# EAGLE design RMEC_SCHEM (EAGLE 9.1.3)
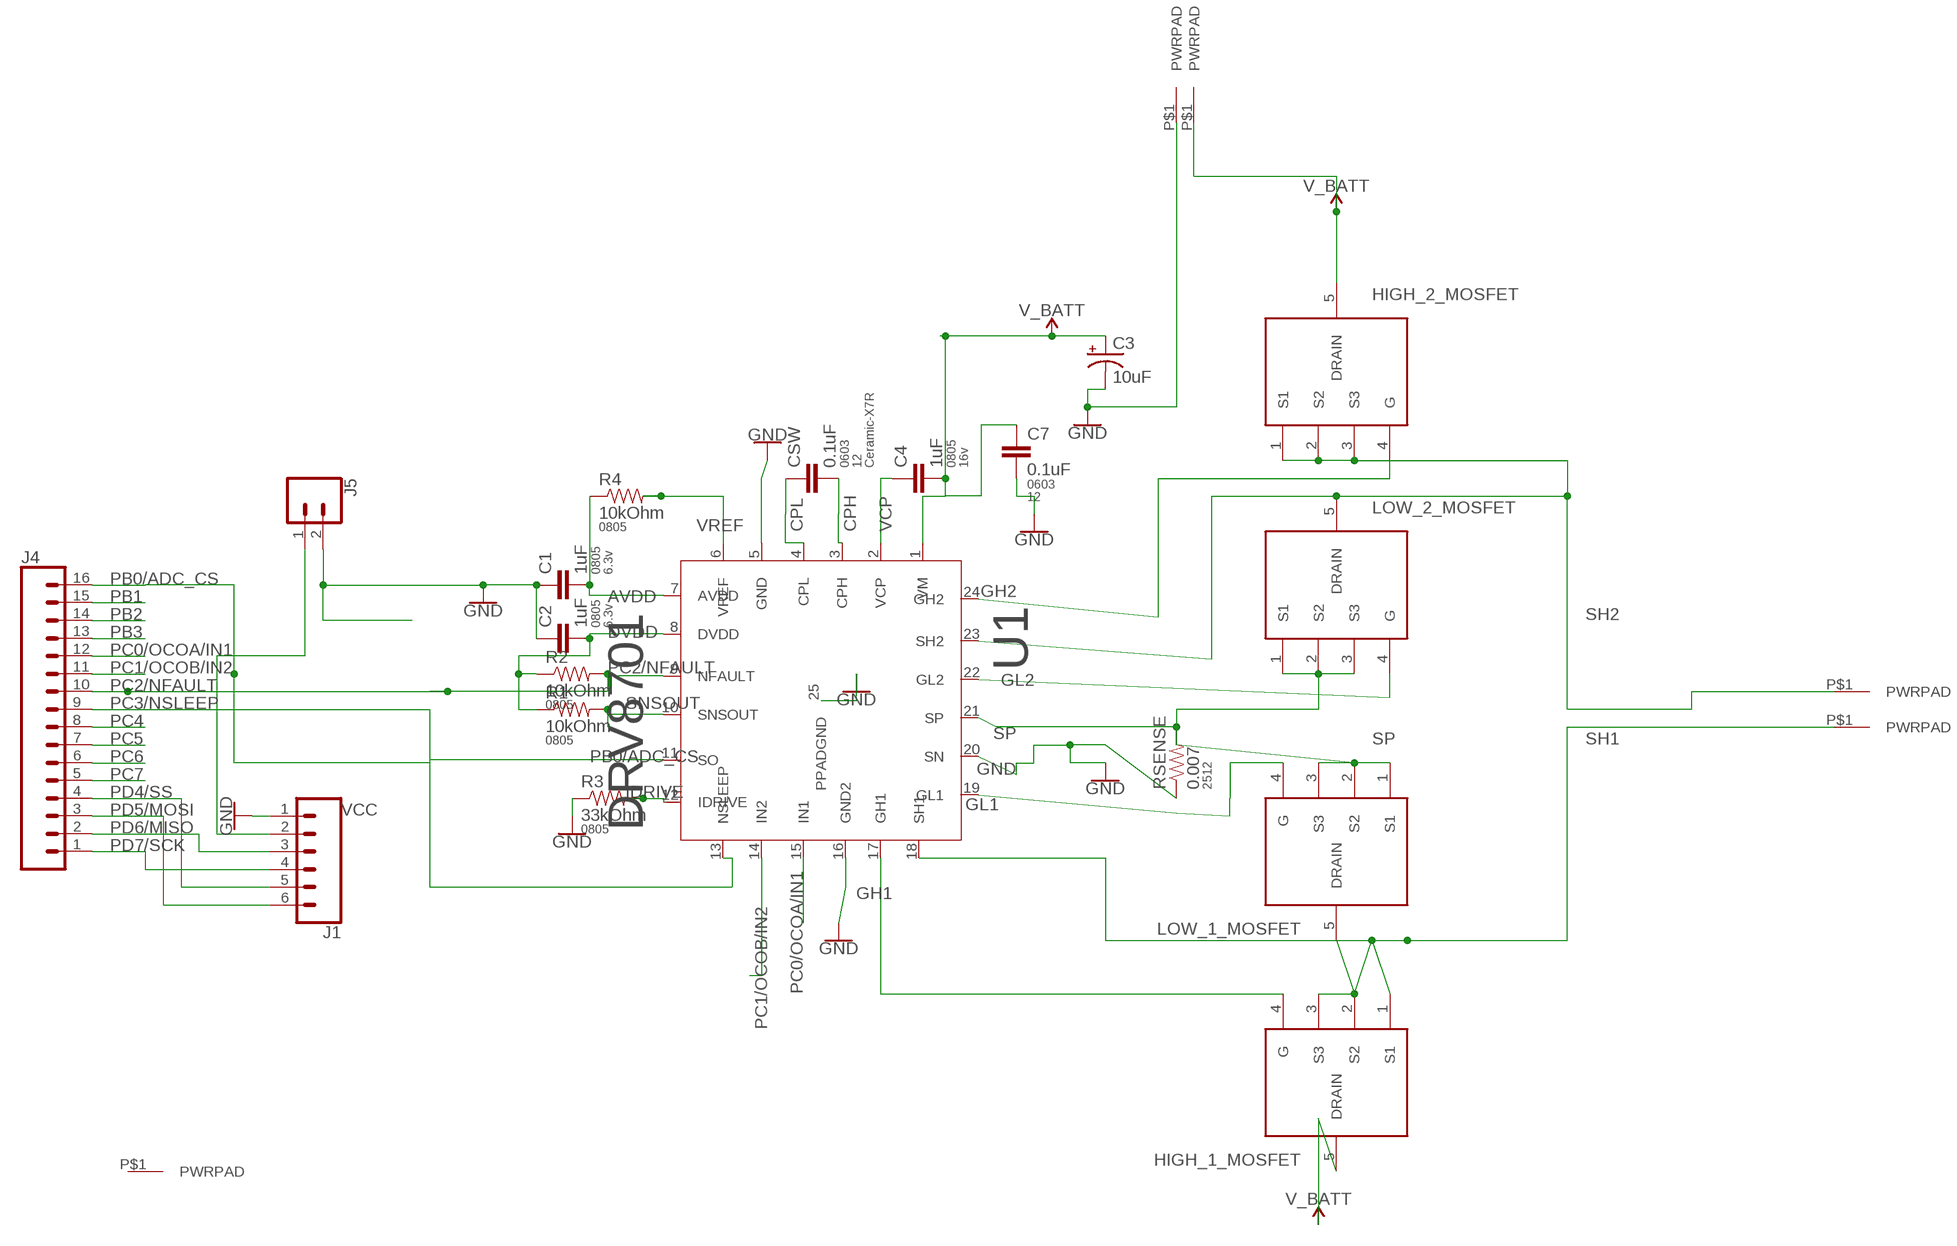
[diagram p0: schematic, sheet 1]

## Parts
C1  1uF  CAP0805  [0805]
C2  1uF  CAP0805  [0805]
C3  10uF  10UF-POLAR-RADIAL-2.5MM-25V-20%  [CPOL-RADIAL-2.5MM-5MM]
C4  1uF  CAP0805  [0805]
C7  0.1uF  CAP0603-CAP  [0603-CAP]
CSW  0.1uF  CAP0603-CAP  [0603-CAP]
GND  PWRPADM3-STANDOFF  [PWRPAD_M3_STANDOFF]
HIGH_1_MOSFET  AON7410  [AON7410]
HIGH_2_MOSFET  AON7410  [AON7410]
J1  CONN_06NO_SILK_FEMALE_PTH  [1X06_NO_SILK]
J3  PWRPADM3  [PWRPAD_3-25MM]
J4  CONN_16  [1X16]
J5  CONN_02  [1X02]
J6  PWRPADM3-STANDOFF  [PWRPAD_M3_STANDOFF]
J7  PWRPADM3-STANDOFF  [PWRPAD_M3_STANDOFF]
LOW_1_MOSFET  AON7410  [AON7410]
LOW_2_MOSFET  AON7410  [AON7410]
R1  10kOhm  RESISTOR0805-RES  [0805]
R2  10kOhm  RESISTOR0805-RES  [0805]
R3  33kOhm  RESISTOR0805-RES  [0805]
R4  10kOhm  RESISTOR0805-RES  [0805]
RSENSE  0.007  RESISTOR2512  [R2512]
U1  DRV8701  [DRV8701]
VM  PWRPADM3-STANDOFF  [PWRPAD_M3_STANDOFF]

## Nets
AVDD: C1.2 R4.1 U1.7(AVDD)
CPH: CSW.2 U1.3(CPH)
CPL: CSW.1 U1.4(CPL)
DVDD: C2.2 R1.1 R2.1 U1.8(DVDD)
GH1: HIGH_1_MOSFET.4(G) U1.17(GH1)
GH2: HIGH_2_MOSFET.4(G) U1.24(GH2)
GL1: LOW_1_MOSFET.4(G) U1.19(GL1)
GL2: LOW_2_MOSFET.4(G) U1.22(GL2)
GND: C1.1 C2.1 C3.2(-) C7.2 GND.P$1(PWRPAD) J1.1 J5.2 R3.1 RSENSE.1 U1.5(GND) U1.16(GND2) U1.20(SN) U1.25(PPADGND)
IDRIVE: R3.2 U1.12(IDRIVE)
PB0/ADC_CS: J4.16 U1.11(SO)
PB1: J4.15
PB2: J4.14
PB3: J4.13
PC0/OCOA/IN1: J4.12 U1.15(IN1)
PC1/OCOB/IN2: J4.11 U1.14(IN2)
PC2/NFAULT: J4.10 R2.2 U1.9(NFAULT)
PC3/NSLEEP: J4.9 U1.13(NSLEEP)
PC4: J4.8
PC5: J4.7
PC6: J4.6
PC7: J4.5
PD4/SS: J1.5 J4.4
PD5/MOSI: J1.6 J4.3
PD6/MISO: J1.3 J4.2
PD7/SCK: J1.4 J4.1
SH1: HIGH_1_MOSFET.1(S1) HIGH_1_MOSFET.2(S2) HIGH_1_MOSFET.3(S3) J7.P$1(PWRPAD) LOW_1_MOSFET.5(DRAIN) U1.18(SH1)
SH2: HIGH_2_MOSFET.1(S1) HIGH_2_MOSFET.2(S2) HIGH_2_MOSFET.3(S3) J6.P$1(PWRPAD) LOW_2_MOSFET.5(DRAIN) U1.23(SH2)
SNSOUT: R1.2 U1.10(SNSOUT)
SP: LOW_1_MOSFET.1(S1) LOW_1_MOSFET.2(S2) LOW_1_MOSFET.3(S3) LOW_2_MOSFET.1(S1) LOW_2_MOSFET.2(S2) LOW_2_MOSFET.3(S3) RSENSE.2 U1.21(SP)
V_BATT: C3.1(+) C4.2 C7.1 HIGH_1_MOSFET.5(DRAIN) HIGH_2_MOSFET.5(DRAIN) U1.1(VM) VM.P$1(PWRPAD)
VCC: J1.2 J5.1
VCP: C4.1 U1.2(VCP)
VREF: R4.2 U1.6(VREF)
Unconnected: J3.P$1(PWRPAD)

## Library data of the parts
C1 C2 = passives:CAP: Capacitor; PACKAGE: 0805; VOLTAGE: 6.3v
C3 = SparkFun-Capacitors:10UF-POLAR: 10.0µF polarized capacitors; PROD_ID: CAP-08440
C4 = passives:CAP: Capacitor; PACKAGE: 0805; VOLTAGE: 16v
C7 = passives:CAP: Capacitor; PACKAGE: 0603; VOLTAGE: 12
CSW = passives:CAP: Capacitor; PACKAGE: 0603; TYPE: Ceramic-X7R; VOLTAGE: 12
GND J3 J6 J7 VM = power:PWRPAD
HIGH_1_MOSFET HIGH_2_MOSFET LOW_1_MOSFET LOW_2_MOSFET = RCustom:AON7410
J1 = SparkFun-Connectors:CONN_06: Multi connection point. Often used as Generic Header-pin footprint for 0.1 inch spaced/style header connections On any of the 0.1 inch spaced packages, you can populate with these: Break Away Headers - Straight (PRT-00116) Break Away Male Headers - Right Angle (PRT-00553) Female Headers (PRT-00115)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; PROD_ID: CONN-08437
J4 = SparkFun-Connectors:CONN_16: Multi connection point. Often used as Generic Header-pin footprint for 0.1 inch spaced/style header connections On any of the 0.1 inch spaced packages, you can populate with these: Break Away Headers - Straight (PRT-00116) Break Away Male Headers - Right Angle (PRT-00553) Female Headers (PRT-00115)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
J5 = SparkFun-Connectors:CONN_02: Multi connection point. Often used as Generic Header-pin footprint for 0.1 inch spaced/style header connections
R1-R4 = passives:RESISTOR: Resistor; PACKAGE: 0805
RSENSE = passives:RESISTOR: Resistor; PACKAGE: 2512
U1 = RCustom:DRV8701: This is the DRV8701, one of TI's gate drivers to make a full bridge for motor control. Includes current sense logic inside with an external sense resistor.

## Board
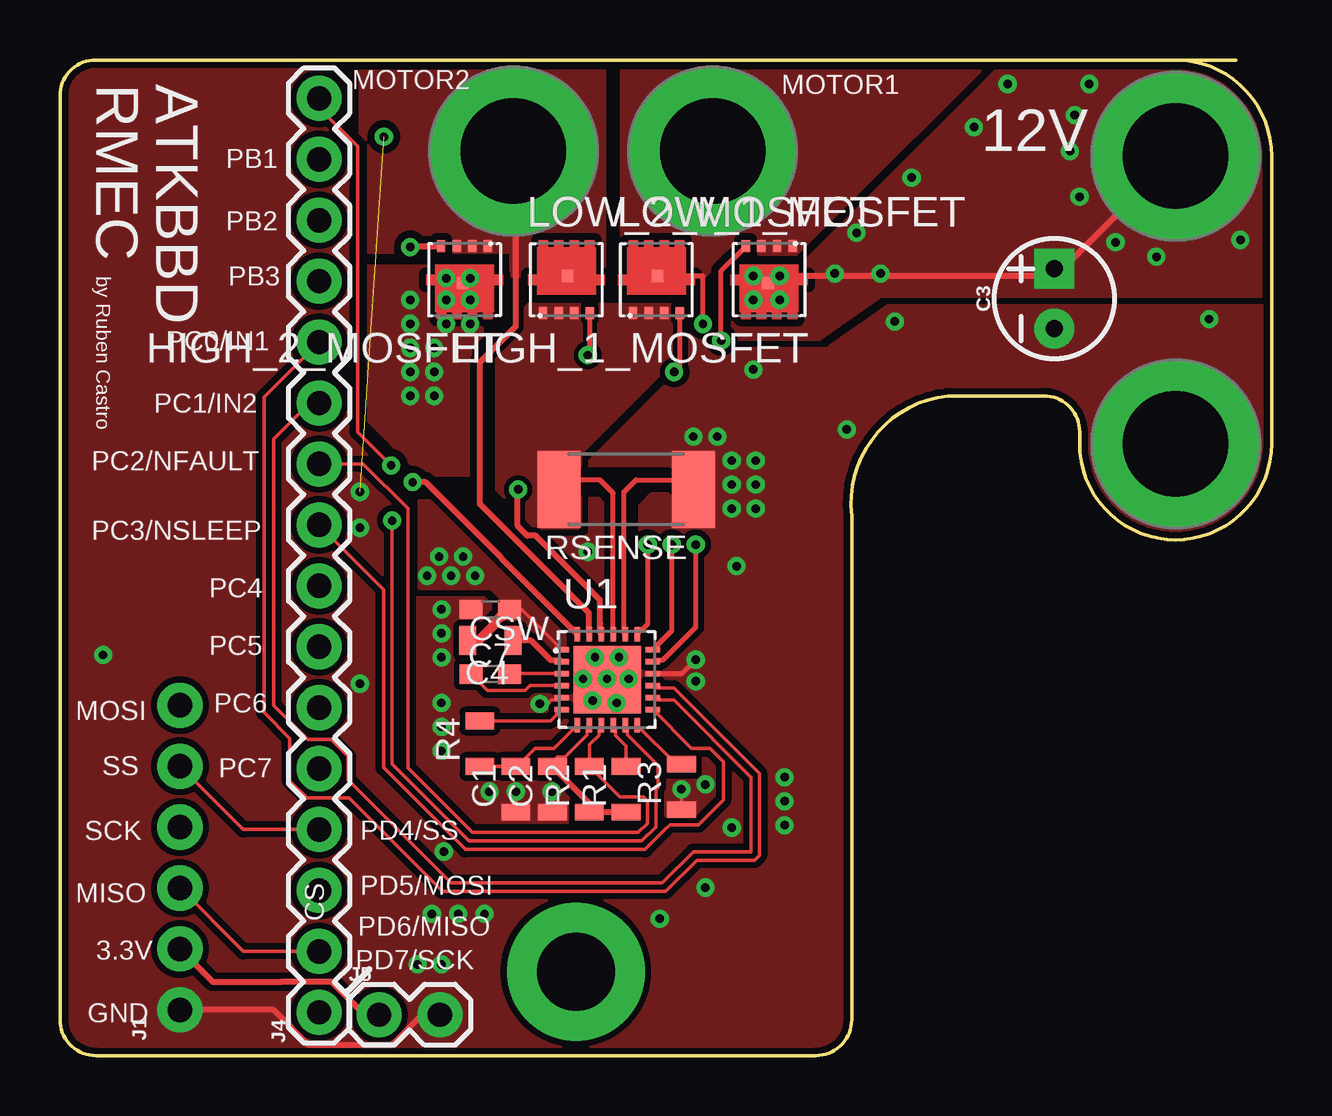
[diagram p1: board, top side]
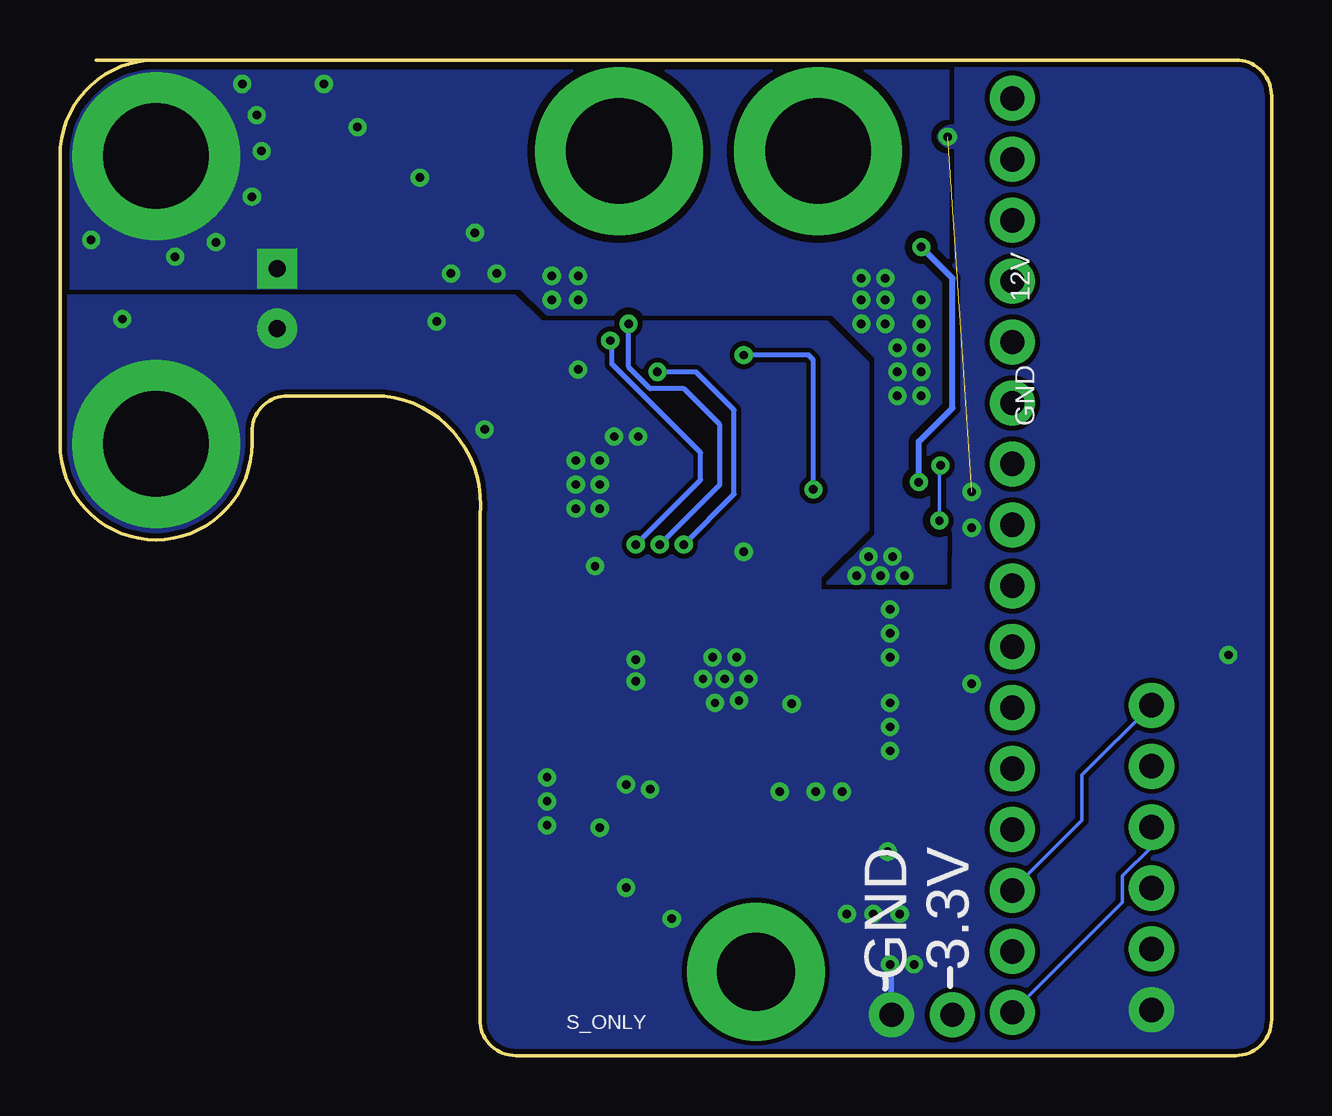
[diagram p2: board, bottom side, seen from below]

Size 50.5 x 41.5 mm. Coordinates in mm from the lower left corner, seen from the top.
Outline: 46.5,41.5 arc-90 50.5,37.5 50.5,25.5 arc-90 46.5,21.5 arc-90 42.5,25.5 42.5,26 arc90 41,27.5 37,27.5 arc90 33,22.5 33,1.5 arc-90 31.5,0 1.5,0 arc-90 0,1.5 0,40 arc-90 1.5,41.5 49,41.5
Copper layers (1*16): Top 0.035mm / dielectric 1.5mm / Bottom 0.035mm
Design rules "default *": minimum track width 6mil, minimum drill 0.35mm, track to track 8mil, track to pad 8mil, pad to pad 8mil, via to via 8mil, smd to smd 8mil, copper to edge 8mil, drill to drill 8mil, minimum pad ring 10mil, minimum via ring 8mil, stop-mask expansion 4mil, vias tented up to drill 25mil, thermal gap 10mil

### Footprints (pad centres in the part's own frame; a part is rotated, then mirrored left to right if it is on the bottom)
0805 = smd 0.7 x 1.2: 1 -0.95,0; 2 0.95,0
CPOL-RADIAL-2.5MM-5MM = drill 0.7 pad 1.651 square: 1 1.25,0 | drill 0.7 pad 1.651: 2 -1.25,0
0603-CAP = smd 0.96 x 0.8: 1 -0.8,0; 2 0.8,0
PWRPAD_M3_STANDOFF = drill 4.4 pad 7: P$1 0,0
AON7410 = smd 0.35 x 0.5: 1 -0.975,-1.4; 2 -0.325,-1.4; 3 0.325,-1.4; 4 0.975,-1.4 | smd 0.5 x 0.5: 5 0.05,0.15
1X06_NO_SILK = drill 1.016 pad 1.88: 1 0,0; 2 2.54,0; 3 5.08,0; 4 7.62,0; 5 10.16,0; 6 12.7,0
PWRPAD_3-25MM = drill 3.25 pad 5.75: P$1 0,0
1X16 = drill 1.016 pad 1.88: 1 0,0; 2 2.54,0; 3 5.08,0; 4 7.62,0; 5 10.16,0; 6 12.7,0; 7 15.24,0; 8 17.78,0; 9 20.32,0; 10 22.86,0; 11 25.4,0; 12 27.94,0; 13 30.48,0; 14 33.02,0; 15 35.56,0; 16 38.1,0
1X02 = drill 1.016 pad 1.88: 1 0,0; 2 2.54,0
R2512 = smd 1.8 x 3.2: 1 -2.8,0; 2 2.8,0
DRV8701 = smd 0.6 x 0.24: 1 -1.9,1.25; 2 -1.9,0.75; 3 -1.9,0.25; 4 -1.9,-0.25; 5 -1.9,-0.75; 6 -1.9,-1.25; 13 1.9,-1.25; 14 1.9,-0.75; 15 1.9,-0.25; 16 1.9,0.25; 17 1.9,0.75; 18 1.9,1.25 | smd 0.24 x 0.6: 7 -1.25,-1.9; 8 -0.75,-1.9; 9 -0.25,-1.9; 10 0.25,-1.9; 11 0.75,-1.9; 12 1.25,-1.9; 19 1.25,1.9; 20 0.75,1.9; 21 0.25,1.9; 22 -0.25,1.9; 23 -0.75,1.9; 24 -1.25,1.9 | smd 2.8 x 2.8: 25 0,0

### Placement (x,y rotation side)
C1  19,11.1 90 top
C2  20.53,11.1 90 top
C3  41.45,31.55 90 top
C4  17.94,17.3 180 top
C7  17.94,18.6 180 top
CSW  17.94,15.9 0 top
GND  46.5,25.5 0 top
HIGH_1_MOSFET  29.56,32.34 180 top
HIGH_2_MOSFET  16.86,32.34 180 top
J1  5,1.9 90 top
J3  21.5,3.5 0 top
J4  10.8,1.8 90 top
J5  13.3,1.7 0 top
J6  18.9,37.7 0 top
J7  27.2,37.7 0 top
LOW_1_MOSFET  24.86,32.34 0 top
LOW_2_MOSFET  21.11,32.34 0 top
R1  23.6,11.1 90 top
R2  22.07,11.1 90 top
R3  25.9,11.2 90 top
R4  17.5,13 90 top
RSENSE  23.6,23.6 180 top
U1  22.81,15.67 0 top
VM  46.5,37.5 0 top

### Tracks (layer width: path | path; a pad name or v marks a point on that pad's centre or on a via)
AVDD
  Top 0.152: U1.7 20.59,12.8 19.8,12.8 19.05,12.05 C1.2 R4.1
CLEAR
  cutout Top (isolate 0.305, no thermals): 22.8,17.5 23.6,17.5 24,17.9 24,23 24.6,23.6 25.4,23.6 25.5,23.5 25.5,24.3 25.4,24.4 21.7,24.4 21.7,23.7 21.7,23.4 22.5,23.4 22.8,23.1
CPH
  Top 0.152: U1.3 18.76,15.92 CSW.2
CPL
  Top 0.152: U1.4 19.59,15.42 19.4,15.22 17.82,15.22 CSW.1
CUTOFFGND
  cutout Top (rank 3, no thermals): 23.8,17.3 23.3,17.3 23.3,17.1 23.8,17.1
DVDD
  Top 0.152: C2.2 20.53,12.24 20.73,12.44 21.05,12.44 21.96,13.35 21.96,13.67 U1.8
  Top 0.254: C2.2 22.07,10.52 R2.1 R1.1
GH1  (via drill 0.35)
  Top 0.203: U1.17 24.79,16.5 25.14,16.5 26.5,17.86 v26.5,21.3 | v27.56,29.8 27.56,32.72 HIGH_1_MOSFET.4
  Bottom 0.203: v27.56,29.8 27.5,29.8 27.5,28.82 23.8,25.12 23.8,24 v26.5,21.3
GH2  (via drill 0.35)
  Top 0.254: U1.24 15.23,23.9 v14.7,23.9 | v14.6,33.7 14.64,33.74 HIGH_2_MOSFET.4
  Bottom 0.254: v14.7,23.9 14.7,25.6 13.3,27 13.3,32.4 v14.6,33.7
GL1  (via drill 0.35)
  Top 0.203: U1.19 24.5,18.01 v24.5,21.3 | v25.6,28.5 25.84,28.73 LOW_1_MOSFET.4
  Bottom 0.203: v24.5,21.3 22.4,23.4 22.4,26.9 24,28.5 v25.6,28.5
GL2  (via drill 0.35)
  Top 0.203: v22,29.2 22.09,29.29 LOW_2_MOSFET.4
  Top 0.254: U1.22 22.52,17.61 22.52,18 22.5,18.02 22.5,19 19.83,21.67 19.48,21.67 19.07,22.07 19.07,23.57 v19.1,23.6
  Bottom 0.203: v19.1,23.6 19.1,29 19.3,29.2 v22,29.2
GND  (via drill 0.35)  (1 unrouted)
  Top 0.152: U1.20 23.5,17.63 | C1.1 v19,11 | C2.1 20.5,10.18 v20.5,11 | v25.9,11.1 R3.1 | U1.5 20.81,14.82 20.49,14.82 20.34,14.66 v20,14.66
  Top 0.2: 24,24 26,24 RSENSE.1
  Top 0.203: 23.5,17.63 23.5,23.5 24,24 | U1.16 25.92,15.92 v26.5,16.5
  Top 0.254: J5.2 15.64,1.9 15.3,1.9 13.83,0.43 10.37,0.43 8.9,1.9 J1.1
  Bottom 0.254: J5.2 15.84,3.74 v15.9,3.8
  other vias: 21.8,15.7 22.2,14.8 23.2,14.7 23.7,15.7 22.8,15.7 22.3,16.6 23.3,16.6 15.9,18.6 26.4,25.8 27.4,25.8 28,24.8 29,24.8 28,23.8 29,23.8 28,22.8 29,22.8 15.5,5.9 16.6,5.9 17.7,5.9 14.9,3.8 17.9,11 15.9,16.6 15.9,17.6 26.9,11.3 30.2,11.6 30.2,10.6 30.2,9.6 26.5,15.6 15.9,14.7 15.9,13.7 15.9,12.7 22,21 28,9.5 16,8.5 12.5,15.5 12.5,22 12.5,23.5 34.8,30.6 47.9,30.7 32.8,26.1 28.9,28.6 26.9,7 28.2,20.4 25,5.7 1.8,16.7 13.5,38.3
  pour Bottom (rank 3, no thermals): -1,54 -4.5,50.5 -4.5,-0.5 -1,-4 35,-4 55.5,16.5 56.5,16.5 56.5,53 0,53
  pour Top (isolate 0.254, rank 3, no thermals): -5.9,52.2 -5.9,-0.7 -0.5,-6.1 35.5,-6.1 58.1,16.5 58.1,52.7 58,52.8 56.3,54.5 -3.8,54.5 -5.9,52.4
IDRIVE
  Top 0.152: R3.2 25.68,12.15 U1.12
PB0/ADC_CS  (via drill 0.35)
  Top 0.152: U1.11 23.66,13.67 23.66,13.35 24.92,12.09 24.92,11.18 24.84,11.1 24.84,9.54 24.24,8.94 17.05,8.94 13.84,12.15 v13.84,22.3 | J4.16 10.8,39.5 12.4,37.9 12.4,26 v13.8,24.6
  Bottom 0.152: v13.84,22.3 13.84,24.56 v13.8,24.6
PC0/OCOA/IN1
  Top 0.152: U1.15 24.81,15.32 25.59,15.32 29.16,11.75 29.16,8.35 28.95,8.14 26.55,8.14 25.25,6.84 15.96,6.84 12.06,10.74 10.29,10.74 9.58,11.46 9.58,13.22 8.5,14.3 8.5,27.44 J4.12
PC1/OCOB/IN2
  Top 0.152: U1.14 24.81,14.82 25.58,14.82 28.8,11.6 28.8,8.5 26.4,8.5 25.1,7.2 16.3,7.2 12.02,11.48 12.02,12.46 11.3,13.18 10.32,13.18 8.9,14.6 8.9,25.7 10.4,27.2 J4.11
PC2/NFAULT
  Top 0.152: U1.9 22.46,13.67 22.46,13.35 22.07,12.96 R2.2 23.34,10.78 24.32,10.78 24.48,10.62 24.48,9.68 24.09,9.3 17.2,9.3 14.5,12 14.5,22.8 12.64,24.66 J4.10
PC3/NSLEEP
  Top 0.152: J4.9 13.49,19.43 13.49,12.01 16.91,8.59 24.39,8.59 25.2,9.4 25.42,9.62 26.62,9.62 27.65,10.65 27.65,12.25 27.1,12.8 26.33,12.8 U1.13
PD4/SS
  Top 0.152: J4.4 7.64,9.42 J1.5
PD5/MOSI
  Bottom 0.152: J1.6 7.9,11.7 7.9,9.8 10.8,6.9 J4.3
PD6/MISO
  Top 0.152: J4.2 7.64,4.34 J1.3
PD7/SCK
  Bottom 0.152: J4.1 6.22,6.38 6.22,7.49 5,8.7 J1.4
SH1  (via drill 0.35)
  Top 0.203: U1.18 25.5,17.71 v25.5,21.3 | v26.8,30.5 26.8,32.49 LOW_1_MOSFET.5
  Bottom 0.203: v26.8,30.5 26.8,28.7 25.9,27.8 24.5,27.8 23,26.3 23,23.8 v25.5,21.3
  pour Top (isolate 0.305, no thermals): 23.4,31.8 26.2,31.8 27.8,33.4 30.7,33.4 40.5,43.2 40.5,44 23.4,44
SH2
  Top 0.254: J6.P$1 19,37.6 19,30.4 17.5,28.9 17.5,23 22.04,18.46 22.04,17.83 22.06,17.81 U1.23
  pour Top (isolate 0.305, no thermals): 18.8,32.5 18.8,33.5 12.5,33.5 12.5,44 22.7,44 22.7,31.9 20.8,31.9 20.8,32.5
SNSOUT
  Top 0.152: R1.2 23.6,12.91 23.16,13.35 23.16,13.67 U1.10
SP
  Top 0.203: U1.21 23.06,23.44 22.5,24 21.2,24 RSENSE.2
  pour Top (no thermals): 19.8,22 21.6,22 21.7,22.1 21.7,25.1 22.1,25.5 26.1,29.5 26.1,31.3 19.5,31.3 19.4,31.2 18.2,30 18.2,27 18.2,23.6
V_BATT  (via drill 0.35)
  Top 0.152: U1.1 19.23,18.6 C7.1
  Top 0.254: VM.P$1 41.8,32.8 C3.1 41.15,32.5 v30,32.5 29.69,32.19 HIGH_1_MOSFET.5
  Top 0.406: C4.2 17.44,17.3 18.13,17.99 18.13,18.07 18.37,18.31 18.45,18.31 C7.1
  other vias: 17.3,20 15.8,20.8 14.6,31.5 14.6,30.5 16.1,30.5 16.1,31.5 17.1,30.5 17.1,31.5 16.1,32.4 17.1,32.4 15.3,20 16.3,20 16.8,20.8 28.9,32.5 28.9,31.5 30,31.5 14.6,29.5 15.6,29.5 15.6,28.5 14.6,28.5 15.6,27.5 14.6,27.5 33.2,34.3 32.3,32.6 35.5,36.6 44,33.9 39.5,40.5 42.9,40.5 42.3,39.2 42.1,37.7 42.5,35.8 45.7,33.3 49.2,34 38.1,38.7 34.2,32.6
  pour Bottom (isolate 0.305, no thermals): 51.5,32 51.5,44.5 13.5,44.5 13.5,32.5 13.6,19.7 18.5,19.7 16.5,21.7 16.5,24 16.5,29.1 18.3,30.9 30.2,30.9 31.3,32 36,32 46.5,32
  pour Top (isolate 0.305, no thermals): 12.5,32.9 17.6,32.9 17.6,30 17.1,29.5 17.1,24.2 15.1,24.2 12.5,26.8
  pour Top (no thermals): 21,17 20.5,17 19.5,18 18.5,18 18.5,19 18,19.5 15,19.5 15,23.1 15.4,23.1 19.5,19 21,17.5
  pour Top (isolate 0.305, no thermals): 28,29.9 31.68,29.9 34.23,31.7 51,31.7 51,45.5 41.5,45.5 41.5,43.5 31,33 28,33
VCC
  Top 0.254: J5.1 12.7,1.7 11.33,3.07 9.2,3.07 6.37,3.07 J1.2
VCP
  Top 0.254: U1.2 20.86,16.47 20.47,16.47 19.64,17.3 C4.1
VREF
  Top 0.152: R4.2 20.44,13.95 U1.6

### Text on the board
tPlace: MOTOR2 | MOTOR1 | RMEC | ATKBBD | 12V | PB1 | PB2 | by Ruben Castro | PB3 | PC0/IN1 | PC1/IN2 | PC2/NFAULT | PC3/NSLEEP | PC4 | PC5 | MOSI | PC6 | SS | PC7 | SCK | PD4/SS | MISO | PD5/MOSI | CS | PD6/MISO | 3.3V | PD7/SCK | GND
bPlace: 12V | GND | 3.3V | GND | S_ONLY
